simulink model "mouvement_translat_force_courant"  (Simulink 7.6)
settings: Solver=ode15s  StartTime=0.0  StopTime=6  RelTol=1e-3
StopFcn:
  | close all
  | load force_courant.mat
  | plot(fi(1,:),fi(2,:),fi(1,:),fi(3,:))
  | axis([0 6 -0.05 0.3])
  | xlabel('temps')
  | title('Force sur l''arbre et courant d''induit')
  | grid
libraries: fl_lib x8, nesl_utility x4, elec_lib x1

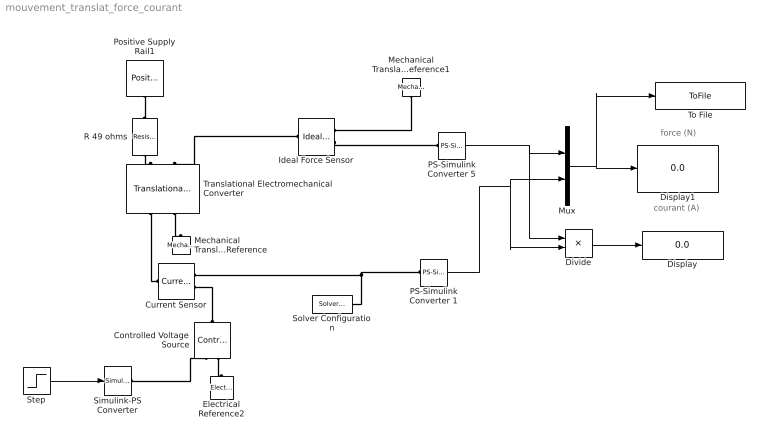
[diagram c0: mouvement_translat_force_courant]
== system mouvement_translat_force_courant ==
  note: force (N)
  note: courant (A)
  Controlled Voltage Source : fl_lib/Electrical/Electrical Sources/Controlled Voltage Source  DialogController=NetworkEngine.DynNeDlgSource  SystemSampleTime=-1  i_Log=off  v_Log=off  LocalVarNames=|i|v  LocalVarDescs=|i|v  LocalVarLogging=[0 0]
  Current Sensor : fl_lib/Electrical/Electrical Sensors/Current Sensor  DialogController=NetworkEngine.DynNeDlgSource  SystemSampleTime=-1  i1_Log=off  v1_Log=off  LocalVarNames=|i1|v1  LocalVarDescs=|i1|v1  LocalVarLogging=[0 0]
  Display : Display
  Display1 : Display
  Divide : Product  Inputs=*/
  Electrical Reference2 : fl_lib/Electrical/Electrical Elements/Electrical Reference  DialogController=NetworkEngine.DynNeDlgSource  SystemSampleTime=-1  i_Log=off  LocalVarNames=|i  LocalVarDescs=|i  LocalVarLogging=[]
  Ideal Force Sensor : fl_lib/Mechanical/Mechanical Sensors/Ideal Force Sensor  DialogController=NetworkEngine.DynNeDlgSource  SystemSampleTime=-1  v_Log=off  f_Log=off  LocalVarNames=|v|f  LocalVarDescs=|v|f  LocalVarLogging=[0 0]
  Mechanical Translational Reference : fl_lib/Mechanical/Translational Elements/Mechanical Translational Reference  DialogController=NetworkEngine.DynNeDlgSource  SystemSampleTime=-1  f_Log=off  LocalVarNames=|f  LocalVarDescs=|f  LocalVarLogging=0
  Mechanical Translational Reference1 : fl_lib/Mechanical/Translational Elements/Mechanical Translational Reference  DialogController=NetworkEngine.DynNeDlgSource  SystemSampleTime=-1  f_Log=off  LocalVarNames=|f  LocalVarDescs=|f  LocalVarLogging=0
  Mux : Mux  Inputs=2
  PS-Simulink Converter 1 : nesl_utility/PS-Simulink Converter  DialogController=NetworkEngine.DynNeUtilDlgSource  SystemSampleTime=-1  PhysicalDomain=network_engine_domain  LeftPortType=input  RightPortType=output  SubClassName=ps_output  Unit=A  AffineConversion=off
  PS-Simulink Converter 5 : nesl_utility/PS-Simulink Converter  DialogController=NetworkEngine.DynNeUtilDlgSource  SystemSampleTime=-1  PhysicalDomain=network_engine_domain  LeftPortType=input  RightPortType=output  SubClassName=ps_output  Unit=N  AffineConversion=off
  Positive Supply Rail1 : elec_lib/Sources/Positive Supply Rail  DialogController=NetworkEngine.DynNeDlgSource  SystemSampleTime=-1  v0=12 V  current_Log=off  voltage_Log=off  power_Log=off  LocalVarNames=|current|voltage|power  LocalVarDescs=|Current (A)|Voltage (V)|Power (W)  LocalVarLogging=[0 0 0]
  R 49 ohms : fl_lib/Electrical/Electrical Elements/Resistor  DialogController=NetworkEngine.DynNeDlgSource  SystemSampleTime=-1  R=49 Ohm  i_Log=off  v_Log=off  LocalVarNames=|i|v  LocalVarDescs=|i|v  LocalVarLogging=[0 0]
  Simulink-PS Converter : nesl_utility/Simulink-PS Converter  DialogController=NetworkEngine.DynNeUtilDlgSource  SystemSampleTime=-1  PhysicalDomain=network_engine_domain  LeftPortType=input  RightPortType=output  SubClassName=ps_input  Unit=1  AffineConversion=off  InputFilterTimeConstant=.001  UdotUserProvided=0
  Solver Configuration : nesl_utility/Solver Configuration  DialogController=NetworkEngine.DynNeUtilDlgSource  SystemSampleTime=-1  PhysicalDomain=network_engine_domain  LeftPortType=input  RightPortType=generic  SubClassName=solver  Accelerate=off  Profile=off  ResidualTolerance=1e-9  MaxNonlinIter=12  MaxModeIter=2  DoFixedCost=off  UseLocalSampling=off  DoDC=off  LinearAlgebra=Sparse  LocalSolverSampleTime=.001  LocalSolverChoice=NE_BACKWARD_EULER_ADVANCER  UseLocalSolver=off
  Step : Step  Before=12  After=0  SampleTime=0
  To File : ToFile  Filename=force_courant.mat  MatrixName=fi
  Translational Electromechanical Converter : fl_lib/Electrical/Electrical Elements/Translational Electromechanical Converter  DialogController=NetworkEngine.DynNeDlgSource  SystemSampleTime=-1  K=0.1 s*V/m  i_Log=off  v_Log=off  f_Log=off  u_Log=off  LocalVarNames=|i|v|f|u  LocalVarDescs=|i|v|f|u  LocalVarLogging=[0 0 0 0]
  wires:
  PS-Simulink Converter 5/1 -> Mux/1, Divide/1
  PS-Simulink Converter 1/1 -> Mux/2, Divide/2
  Mux/1 -> Display1/1, To File/1
  Divide/1 -> Display/1
  Step/1 -> Simulink-PS Converter/1
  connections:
  Ideal Force Sensor/LConn1 -- Translational Electromechanical Converter/LConn2
  Ideal Force Sensor/RConn2 -- PS-Simulink Converter 5/LConn1
  Translational Electromechanical Converter/RConn2 -- Mechanical Translational Reference/LConn1
  Mechanical Translational Reference1/LConn1 -- Ideal Force Sensor/RConn1
  Positive Supply Rail1/RConn1 -- R 49 ohms/LConn1
  R 49 ohms/RConn1 -- Translational Electromechanical Converter/LConn1
  Translational Electromechanical Converter/RConn1 -- Current Sensor/LConn1
  Current Sensor/RConn1 -- PS-Simulink Converter 1/LConn1 -- Solver Configuration/RConn1
  Controlled Voltage Source/RConn2 -- Electrical Reference2/LConn1
  Simulink-PS Converter/RConn1 -- Controlled Voltage Source/RConn1
  Controlled Voltage Source/LConn1 -- Current Sensor/RConn2
